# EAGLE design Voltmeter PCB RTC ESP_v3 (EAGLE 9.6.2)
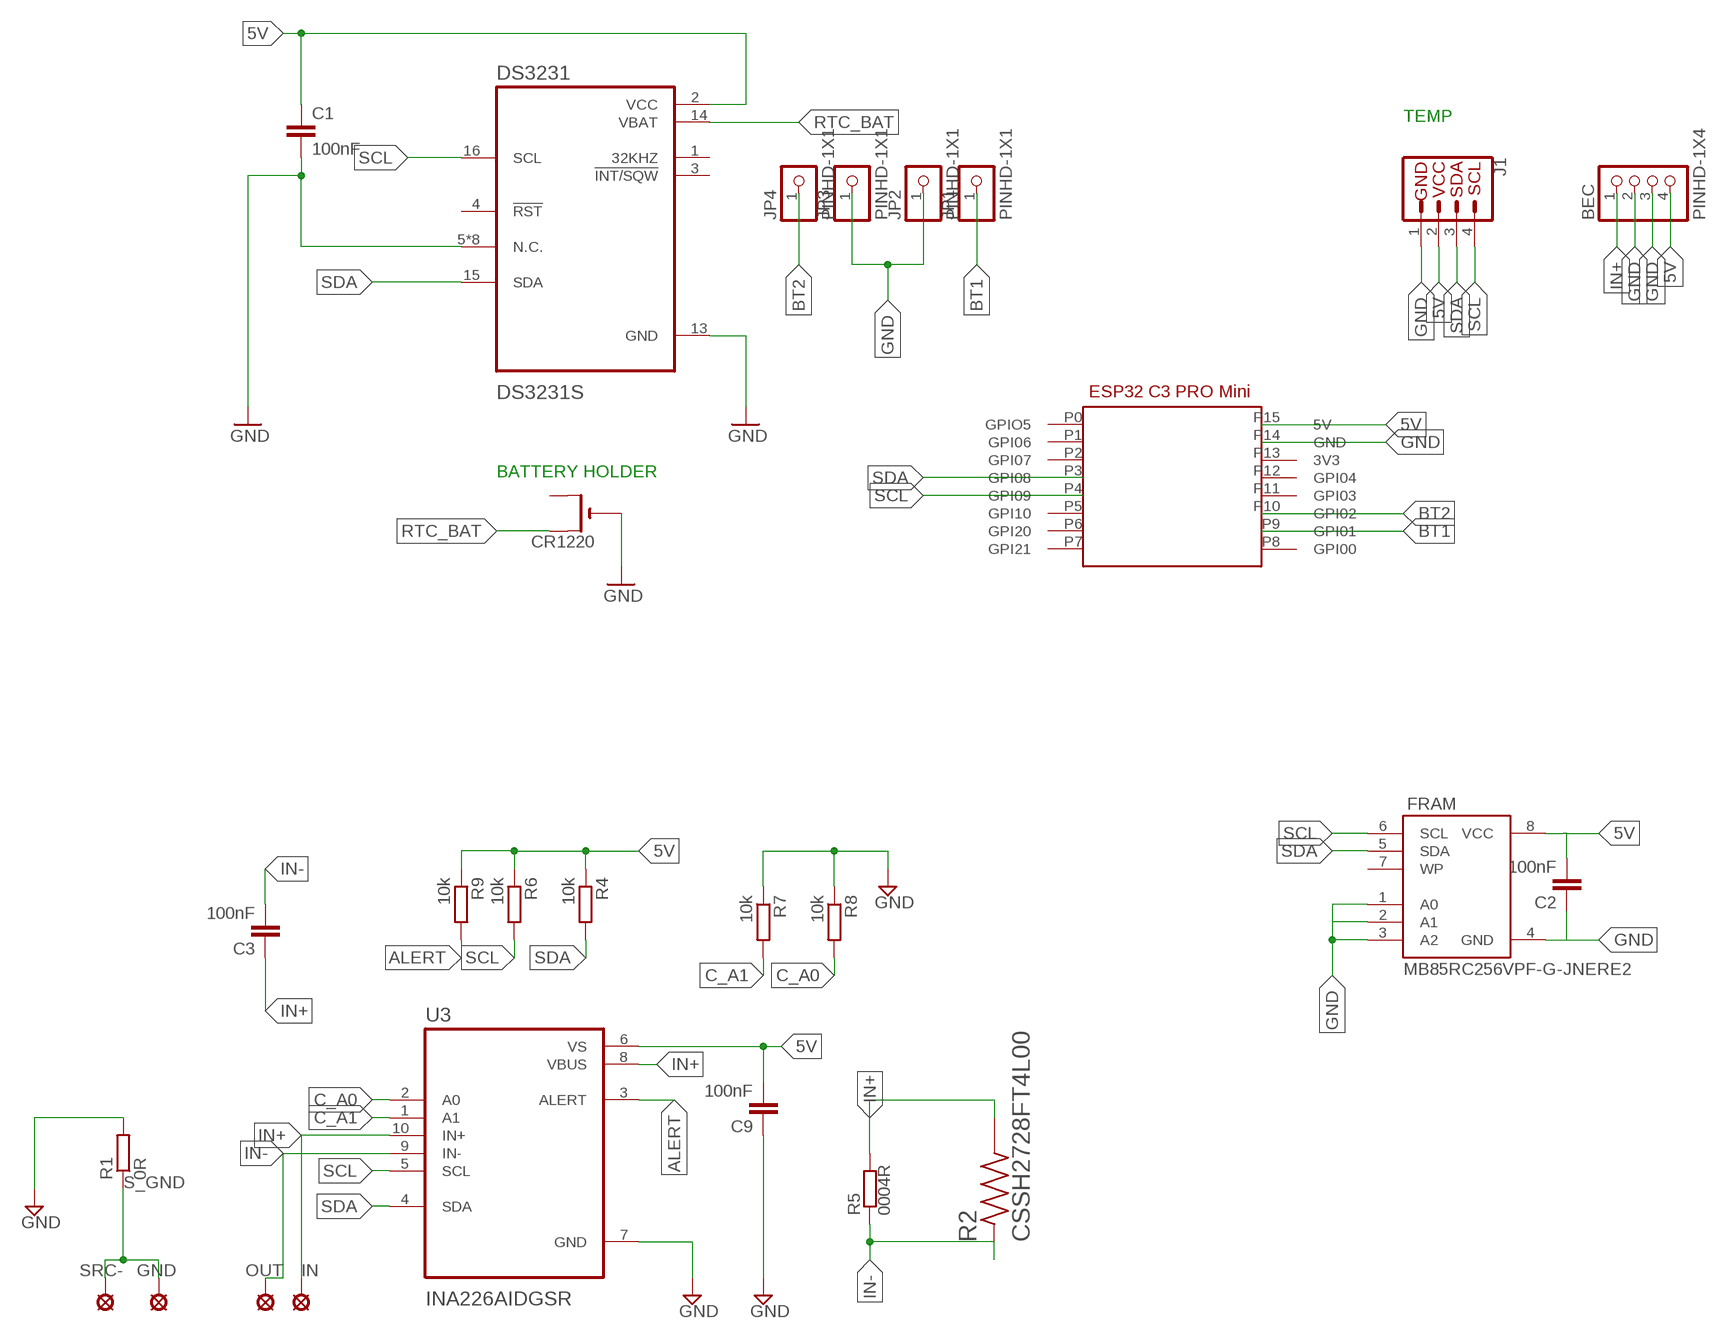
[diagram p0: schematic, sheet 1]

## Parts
BEC  PINHD-1X4  [1X04]
C1  100nF  C-EUC0603  [C0603]
C2  100nF  C-EUC0603  [C0603]
C3  100nF  C-EUC0603  [C0603]
C9  100nF  C-EUC0603  [C0603]
CR1220  CR1220SMT  [CR1220-SMD]
DS3231  DS3231S  [SOIC127P1032X265-16N]
FRAM  MB85RC256VPF-G-JNERE2  [SOIC8_208MIL]
GND  SE14  [SE14]
IN  SE14  [SE14]
J1  QWIIC_CONNECTORJS-1MM  [1X04_1MM_RA]
JP1  PINHD-1X1  [1X01]
JP2  PINHD-1X1  [1X01]
JP3  PINHD-1X1  [1X01]
JP4  PINHD-1X1  [1X01]
OUT  SE14  [SE14]
R1  0R  R-EU_R1206  [R1206]
R2  CSSH2728FT4L00  [RESC6771X124N]
R4  10k  R-EU_R0603  [R0603]
R5  0004R  BVS  [BVS]
R6  10k  R-EU_R0603  [R0603]
R7  10k  R-EU_R0603  [R0603]
R8  10k  R-EU_R0603  [R0603]
R9  10k  R-EU_R0603  [R0603]
SRC-  SE14  [SE14]
U3  INA226AIDGSR  [SOP50P490X110-10N]
U$1  ESP32_C3_PROV1  [ESP32_C2_PRO]

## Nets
5V: BEC.4 C1.1 C2.2 C9.2 DS3231.2(VCC) FRAM.8(VCC) J1.2(VCC) R4.1 R6.1 R9.1 U3.6(VS) U$1.P15(5V)
ALERT: R9.2 U3.3(ALERT)
BT1: JP1.1 U$1.P9(GPI01)
BT2: JP4.1 U$1.P10(GPI02)
C_A0: R8.2 U3.2(A0)
C_A1: R7.2 U3.1(A1)
GND: BEC.2 BEC.3 C1.2 C2.1 C9.1 CR1220.- DS3231.5(N.C.) DS3231.6(N.C.) DS3231.7(N.C.) DS3231.8(N.C.) DS3231.9(N.C.) DS3231.10(N.C.) DS3231.11(N.C.) DS3231.12(N.C.) DS3231.13(GND) FRAM.1(A0) FRAM.3(A2) FRAM.4(GND) J1.1(GND) JP2.1 JP3.1 R1.2 R7.1 R8.1 U3.7(GND) U$1.P14(GND)
IN+: BEC.1 C3.1 IN.MP R2.2 R5.1 U3.8(VBUS) U3.10(IN+)
IN-: C3.2 OUT.MP R2.1 R5.2 U3.9(IN-)
N$2: FRAM.2(A1)
RTC_BAT [medium]: CR1220.+$1(+) DS3231.14(VBAT)
S_GND [high_current]: GND.MP R1.1 SRC-.MP
SCL: DS3231.16(SCL) FRAM.6(SCL) J1.4(SCL) R6.2 U3.5(SCL) U$1.P4(GPI09)
SDA: DS3231.15(SDA) FRAM.5(SDA) J1.3(SDA) R4.2 U3.4(SDA) U$1.P3(GPI08)
Unconnected: CR1220.+$2(+1) DS3231.1(32KHZ) DS3231.3(!INT/SQW) DS3231.4(!RST) FRAM.7(WP) U$1.P0(GPIO5) U$1.P1(GPI06) U$1.P2(GPI07) U$1.P5(GPI10) U$1.P6(GPI20) U$1.P7(GPI21) U$1.P8(GPI00) U$1.P11(GPI03) U$1.P12(GPI04) U$1.P13(3V3)

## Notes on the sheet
- TEMP
- BATTERY HOLDER

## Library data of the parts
BEC = Connector:PINHD-1X4: PIN HEADER; CATEGORY: CONNECTOR; SUB-CATEGORY: PIN-HEADER
C1 = resistor:C-EU: CAPACITOR, European symbol
C2 C3 C9 = rcl:C-EU: CAPACITOR, European symbol; SPICEPREFIX: C
CR1220 = adafruit:CR1220: CR1216/CR1220/CR1225 12mm 3V lithium coin cell Great for battery packup. Both SMT and THM holders. Note the THM package has the ground pads on both sides of the PCB so that the masks are the same - this reduces the cost
DS3231 = DS3231S:DS3231S: Check prices; AVAILABILITY: Warning; DESCRIPTION: Real Time Clock (RTC) IC Clock/Calendar I²C, 2-Wire Serial 16-SOIC (0.295, 7.50mm Width); MF: Maxim Integrated; MP: DS3231S; PACKAGE: SOIC-16 Maxim Integrated; PRICE: None; PURCHASE-URL: https://pricing.snapeda.com/search/part/DS3231S/?ref=eda
FRAM = MB85RC256VPF-G-JNERE2:MB85RC256VPF-G-JNERE2: Check availability; AVAILABILITY: In Stock; CHECK_PRICES: https://www.snapeda.com/parts/MB85RC256VPFGJNERE2/Fujitsu/view-part/?ref=eda; DESCRIPTION: 256 K (32 K × 8) Bit I2C | IC FRAM 256K I2C 1MHZ 8SOP; MF: Fujitsu Semiconductors; MP: MB85RC256VPFGJNERE2; PACKAGE: None; PRICE: None; SNAPEDA_LINK: https://www.snapeda.com/parts/MB85RC256VPFGJNERE2/Fujitsu/view-part/?ref=snap
GND IN OUT SRC- = solpad:SE14: SOLDER PAD
J1 = SparkFun-Connectors:QWIIC_CONNECTOR: SparkFun I2C Standard Qwiic Connector An SMD 1mm pitch JST connector makes it easy and quick (get it? Qwiic?) to connect I2C devices to each other. The Qwiic system enables fast and solderless connection between popular platforms and various sensors and actuators. We carry 200mm, 100mm, 50mm, and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
JP1-JP4 = Connector:PINHD-1X1: PIN HEADER; CATEGORY: CONNECTOR; SUB-CATEGORY: PIN-HEADER
R1 R4 R6-R9 = rcl:R-EU_: RESISTOR, European symbol; SPICEPREFIX: R
R2 = CSSH2728FT4L00:CSSH2728FT4L00: Check availability; AVAILABILITY: In Stock; CHECK_PRICES: https://www.snapeda.com/parts/CSSH2728FT4L00/Stackpole+Electronics/view-part/?ref=eda; DESCRIPTION: 4 mOhms ±1% 4W Chip Resistor Wide 2827 (7067 Metric), 2728 Automotive AEC-Q200, Current Sense Metal Element; MF: Stackpole Electronics Inc; MP: CSSH2728FT4L00; PACKAGE: 6771 Stackpole; PRICE: None; SNAPEDA_LINK: https://www.snapeda.com/parts/CSSH2728FT4L00/Stackpole+Electronics/view-part/?ref=snap
R5 = resistor-shunt:BVS: SMD SHUNT RESISTOR; OC_FARNELL: unknown; OC_NEWARK: unknown
U3 = INA226AIDGSR:INA226AIDGSR: Check availability; AVAILABILITY: In Stock; CHECK_PRICES: https://www.snapeda.com/parts/INA226AIDGSR/Texas+Instruments/view-part/?ref=eda; DESCRIPTION: 36V, 16-bit, ultra-precise i2c output current/voltage/power monitor w/alert; MF: Texas Instruments; MP: INA226AIDGSR; PACKAGE: VSSOP-10 Texas Instruments; PRICE: None; SNAPEDA_LINK: https://www.snapeda.com/parts/INA226AIDGSR/Texas+Instruments/view-part/?ref=snap
U$1 = albert:ESP32_C3_PRO

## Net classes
0 default: width 0.305 mm, drill 0.254 mm, clearance 0.381 mm
1 high_current: width 3 mm, drill 0.508 mm, clearance 0.9 mm
2 medium: width 0.381 mm, drill 0.3 mm, clearance 0.381 mm

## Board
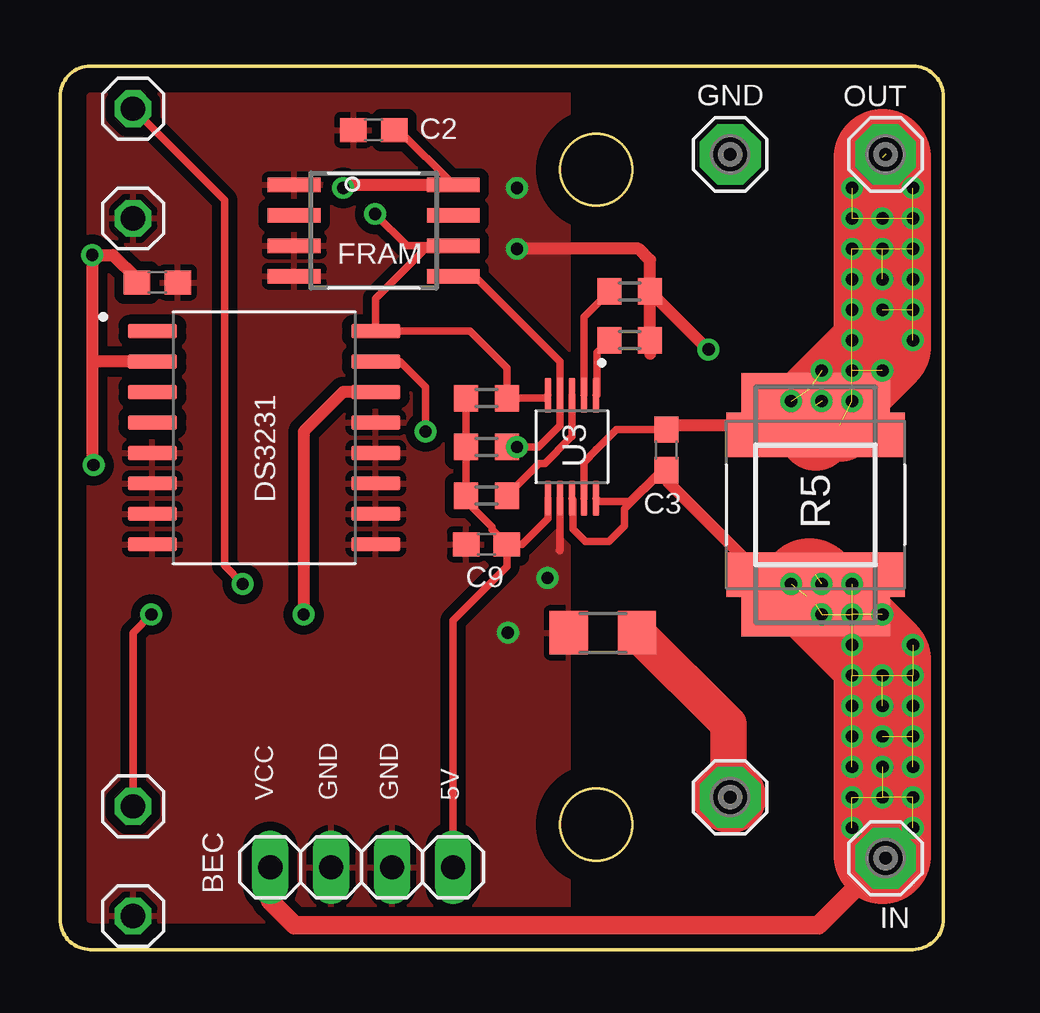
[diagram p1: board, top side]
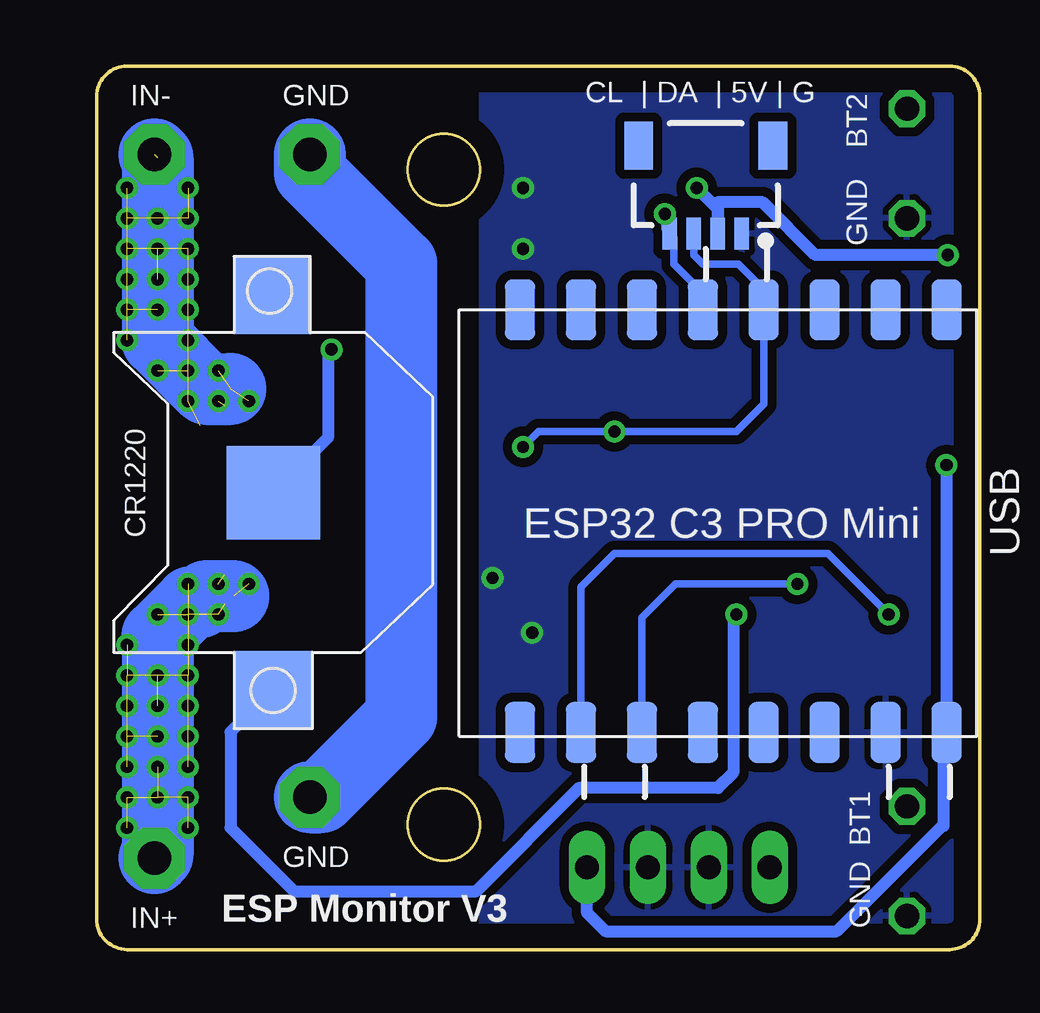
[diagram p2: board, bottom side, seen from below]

Size 36.83 x 36.83 mm. Coordinates in mm from the lower left corner, seen from the top.
Outline: 35.56,0 1.27,0 arc-90 0,1.27 0,35.56 arc-90 1.27,36.83 35.56,36.83 arc-90 36.83,35.56 36.83,1.27 arc-90 35.56,0
Outline: circle at 22.35,32.51 radius 1.5
Outline: circle at 22.35,5.21 radius 1.5
Copper layers (1*16): Top 0.035mm / dielectric 1.5mm / Bottom 0.035mm
Design rules "default *": minimum track width 10mil, minimum drill 0.35mm, track to track 9mil, track to pad 9mil, pad to pad 6mil, via to via 6mil, smd to smd 6mil, copper to edge 40mil, drill to drill 6mil, minimum pad ring 10mil, minimum via ring 8mil, stop-mask expansion 4mil, vias tented up to drill 100mil, thermal gap 10mil

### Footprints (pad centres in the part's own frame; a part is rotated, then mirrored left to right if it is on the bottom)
1X04 = drill 1.016 long: 1 -3.81,0; 2 -1.27,0; 3 1.27,0; 4 3.81,0
C0603 = smd 1.1 x 1: 1 -0.85,0; 2 0.85,0
CR1220-SMD = smd 3.2 x 3.2: +$1 -8.2,0; +$2 8.2,0 | smd 3.9 x 3.9: - 0,0
SOIC127P1032X265-16N = smd 2.05 x 0.59: 1 -4.655,4.445; 2 -4.655,3.175; 3 -4.655,1.905; 4 -4.655,0.635; 5 -4.655,-0.635; 6 -4.655,-1.905; 7 -4.655,-3.175; 8 -4.655,-4.445; 9 4.655,-4.445; 10 4.655,-3.175; 11 4.655,-1.905; 12 4.655,-0.635; 13 4.655,0.635; 14 4.655,1.905; 15 4.655,3.175; 16 4.655,4.445
SOIC8_208MIL = smd 0.6 x 2.2: 1 -1.905,-3.315; 2 -0.635,-3.315; 3 0.635,-3.315; 4 1.905,-3.315; 5 1.905,3.315; 6 0.635,3.315; 7 -0.635,3.315; 8 -1.905,3.315
SE14 = drill 1.397 pad 2.54 octagon: MP 0,0
1X04_1MM_RA = smd 0.6 x 1.35: 1 -1.5,0; 2 -0.5,0; 3 0.5,0; 4 1.5,0 | smd 1.2 x 2: NC1 2.8,-3.675; NC2 -2.8,-3.675
1X01 = drill 1.016 octagon: 1 0,0
R1206 = smd 1.6 x 1.803: 1 -1.422,0; 2 1.422,0
RESC6771X124N = smd 1.84 x 7.45: 1 -2.916,0; 2 2.916,0
R0603 = smd 1 x 1.1: 1 -0.85,0; 2 0.85,0
BVS = smd 2.7 x 6.2: 1 -4.14,0; 2 4.14,0
SOP50P490X110-10N = smd 1.47 x 0.28: 1 -2.15,1; 2 -2.15,0.5; 3 -2.15,0; 4 -2.15,-0.5; 5 -2.15,-1; 6 2.15,-1; 7 2.15,-0.5; 8 2.15,0; 9 2.15,0.5; 10 2.15,1
ESP32_C2_PRO = smd 2.54 x 1.27: P0 -2.54,19.05; P1 -2.54,16.51; P2 -2.54,13.97; P3 -2.54,11.43; P4 -2.54,8.89; P5 -2.54,6.35; P6 -2.54,3.81; P7 -2.54,1.27; P8 15.08,1.27; P9 15.08,3.81; P10 15.08,6.35; P11 15.08,8.89; P12 15.08,11.43; P13 15.08,13.97; P14 15.08,16.51; P15 15.08,19.05

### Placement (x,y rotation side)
BEC  12.57,3.43 0 top
C1  4.06,27.81 0 top
C2  13.08,34.16 0 top
C3  25.27,20.83 90 top
C9  17.78,16.89 0 top
CR1220  29.46,19.05 90 bottom
DS3231  8.51,21.34 0 top
FRAM  13.08,29.97 270 top
GND  27.94,33.15 0 top
IN  34.42,3.81 90 top
J1  11.43,29.84 180 bottom
JP1  3.05,5.97 0 top
JP2  3.05,1.4 0 top
JP3  3.05,30.48 0 top
JP4  3.05,35.05 0 top
OUT  34.42,33.15 0 top
R1  22.63,13.21 180 top
R2  31.5,18.54 270 top
R4  17.78,20.95 0 top
R5  31.5,18.54 90 top
R6  17.78,22.99 0 top
R7  23.75,25.4 180 top
R8  23.75,27.43 180 top
R9  17.78,18.92 0 top
SRC-  27.94,6.35 0 top
U3  21.34,20.95 270 top
U$1  20.45,24.13 270 bottom

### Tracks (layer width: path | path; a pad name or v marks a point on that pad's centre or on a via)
5V  (via drill 0.51)
  Top 0.305: U3.6 20.34,17.96 19.27,16.89 C9.2 | C9.2 18.63,15.96 16.38,13.72 BEC.4 | C2.2 14.11,34.16 FRAM.8 | C9.2 18.01,17.51 18.01,17.61 16.93,18.7 R9.1 R4.1 R6.1
  Top 0.508: 1.35,24.51 v1.35,28.96 2.2,28.96 3.21,27.94 C1.1 | 1.35,24.51 1.35,20.24 v1.4,20.19 | DS3231.2 1.35,24.51 | v11.81,31.75 11.94,31.88 FRAM.8
  Bottom 0.508: BEC.4 16.38,1.52 15.62,0.76 5.97,0.76 1.58,5.15 1.52,5.15 1.52,8.92 U$1.P15 v1.4,20.19 | v1.35,28.96 6.86,28.96 9.06,31.16 10.93,31.16 J1.2 10.93,30.87 v11.81,31.75
ALERT
  Top 0.305: R9.2 19.98,20.27 20.22,20.27 21.25,21.3 21.34,21.38 U3.3
BT1  (via drill 0.51)
  Top 0.305: v3.81,13.97 3.05,13.21 JP1.1
  Bottom 0.305: U$1.P9 16.64,15.11 15.24,16.51 6.35,16.51 v3.81,13.97
BT2  (via drill 0.51)
  Top 0.305: JP4.1 6.86,31.24 6.86,16 v7.62,15.24
  Bottom 0.305: v7.62,15.24 12.7,15.24 14.1,13.84 U$1.P10
C_A0
  Top 0.305: U3.2 21.84,26.37 R8.2
C_A1
  Top 0.305: R7.2 22.38,24.88 22.38,23.11 U3.1
GND  (via drill 0.51)
  Top 0.305: U3.7 20.84,16.64 20.83,16.64
  Top 0.508: R8.1 R7.1 24.6,24.84 | R8.1 24.6,28.74 24.13,29.21 v19.05,29.21 | v27.04,25.02 27.01,25.02 R8.1
  Bottom 0.508: CR1220.- 27.18,21.34 27.18,24.88 v27.04,25.02
  other vias: 19.05,31.75 20.32,15.49 18.67,13.21
  pour Top: -2.54,39.37 -2.54,-2.54 21.21,-2.54 21.21,39.37
  pour Bottom: -2.54,39.37 -2.54,-5.08 20.83,-5.08 20.83,39.37
IN+  (via drill 0.51)  (24 unrouted)
  Top 0.305: C3.1 25.15,19.98 23.53,18.36 23.53,17.66 22.89,17.02 21.91,17.02 21.39,17.53 21.39,18.75 U3.8 | U3.10 22.47,18.67 23.75,18.67 24.89,19.81 25.27,19.81 25.27,19.43 28.7,16 30.99,16 34.29,12.7 34.29,3.94 IN.MP
  Top 0.508: 31.36,15.24 29.59,15.24 25.39,19.44 25.4,19.44 25.4,19.85 C3.1
  Top 0.762: BEC.1 8.76,2.03 9.78,1.02 31.62,1.02 34.29,3.68 34.29,3.94
  Top 1.27: 31.62,15.5 R2.2 | R5.1 31.5,15.37
  Top 3: 31.24,15.12 31.36,15.24 31.5,15.37 31.62,15.5
  Top 4.064: 31.24,15.12 34.29,12.07 v34.29,6.35 34.29,3.94
  Bottom 3: IN.MP 34.29,3.94 34.29,13.08 32.89,14.48 32.51,14.48 32.26,14.73 31.11,14.73
  other vias: 35.56,6.35 33.02,6.35 33.02,7.62 33.02,8.89 33.02,10.16 33.02,11.43 33.02,12.7 31.75,13.97 34.29,7.62 35.56,7.62 34.29,8.89 34.29,10.16 34.29,11.43 35.56,8.89 35.56,10.16 35.56,11.43 35.56,12.7 34.29,13.97 33.02,15.24 33.02,13.97 31.75,15.24 30.48,15.24 35.56,5.08 33.02,5.08
IN-  (via drill 0.51)  (23 unrouted)
  Top 0.305: 22.35,20.82 22.34,20.84 | 22.35,20.82 23.2,21.68 C3.2 25.43,21.84 29.21,21.84 | U3.9 21.84,20.31 22.35,20.82
  Top 0.508: 31.5,21.84 29.21,21.84 25.51,21.84
  Top 1.27: 31.5,21.84 R5.2 31.5,22.35 31.5,21.84
  Top 3: 31.5,21.84 R2.1 31.88,21.84 32.51,21.84
  Top 4.064: 31.5,22.35 34.29,25.15 34.29,33.02
  Bottom 3: OUT.MP 34.29,33.02 34.29,25.4 32.26,23.37 31.24,23.37
  other vias: 35.56,25.4 33.02,25.4 33.02,26.67 33.02,27.94 34.29,26.67 34.29,27.94 34.29,29.21 34.29,30.48 34.29,24.13 33.02,22.86 33.02,24.13 31.75,24.13 31.75,22.86 33.02,29.21 33.02,30.48 35.56,26.67 35.56,27.94 35.56,29.21 35.56,30.48 35.56,31.75 33.02,31.75 30.48,22.86
RTC_BAT  (via drill 0.51)
  Top 0.508: DS3231.14 11.81,23.24 10.16,21.59 v10.16,13.97
  Bottom 0.508: v10.16,13.97 10.29,13.84 10.29,7.37 10.92,6.73 16.72,6.73 21.04,2.41 28.57,2.41 31.24,5.08 31.24,9.07 CR1220.+$1
S_GND
  Top 1.524: R1.1 27.86,9.4 27.86,6.43
  Top 3: SRC-.MP 27.86,6.43
  Bottom 3: GND.MP 27.94,32.38 24.13,28.57 24.13,9.7 27.48,6.35 SRC-.MP
SCL  (via drill 0.51)
  Top 0.305: U3.5 20.22,22.99 R6.2 18.63,24.23 17.08,25.78 DS3231.16 13.16,27.13 15.24,29.21 16.27,29.21 FRAM.6 14.47,29.34 v13.14,30.67
  Bottom 0.305: U$1.P4 11.56,27.36 12.76,28.57 12.76,29.68 J1.4 13.14,30.06 v13.14,30.67
SDA  (via drill 0.51)
  Top 0.305: R4.2 v19.05,20.95 19.94,20.95 20.84,21.85 U3.4 20.84,24.5 17.27,28.07 FRAM.5 | DS3231.15 14.18,24.51 15.24,23.45 v15.24,21.59
  Bottom 0.305: J1.3 11.93,28.96 11.55,28.57 10.07,28.57 9.02,27.52 U$1.P3 9.02,22.73 10.16,21.59 v15.24,21.59 18.41,21.59 v19.05,20.95

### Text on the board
tNames: VCC | GND | GND | 5V
bNames: CL | DA | 5V | G | BT2 | GND | IN- | GND | BT1 | GND | GND | ESP Monitor V3 | IN+

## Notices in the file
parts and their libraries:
SparkFun-Connectors: Licensing: Creative Commons ShareAlike 4.0 International - https://creativecommons.org/licenses/by-sa/4.0
